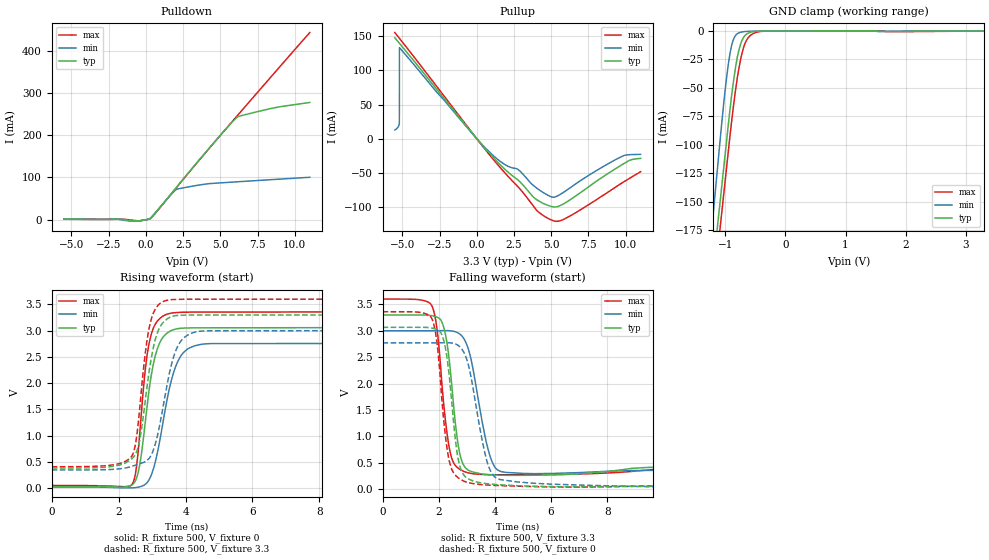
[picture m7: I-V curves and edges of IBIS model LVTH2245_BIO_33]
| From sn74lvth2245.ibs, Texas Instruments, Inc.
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[Model]   LVTH2245_BIO_33
Model_type  I/O
Vinl = 0.8
Vinh = 2.34
Enable   Active-Low
Vref =   0
Rref =   500
Cref =   50p
Vmeas =   1.5
| variable   typ   min   max
C_comp   6.47pF   5.20pF   8.54pF
| C_pullup   4.87pF   3.70pF   5.94pF
| C_pulldown   5.78pF   0.20pF   11.87pF
| C_tri-state   6.47pF   5.20pF   8.54pF
[Temperature Range]   40   -40   100
| Ambient temperature   25   -40   85
[Voltage range]   3.3   3   3.6
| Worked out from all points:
|   slope of the pulldown table from 0 to 0.495 V, typ, clamps not added: 47.8 ohm
|   slope of the pullup table from 0 to 0.495 V, typ, clamps not added: 38.7 ohm
|   GND clamp passes 1 mA (typ) near -0.58 V on its own axis
|   rising waveform, R_fixture 500, V_fixture 0: 20-80 % time 391ps typ, 525ps min, 307ps max; typ from 0.039 V to 3.06 V
|   falling waveform, R_fixture 500, V_fixture 3.3: 20-80 % time 348ps typ, 554ps min, 342ps max; typ from 3.3 V to 0.384 V
|   rising waveform, R_fixture 500, V_fixture 3.3: 20-80 % time 408ps typ, 518ps min, 335ps max; typ from 0.386 V to 3.3 V
|   falling waveform, R_fixture 500, V_fixture 0: 20-80 % time 365ps typ, 582ps min, 358ps max; typ from 3.07 V to 0.039 V
[GND Clamp]
| LVTH2245_BIO_33
|   Voltage   I(typ)   I(min)   I(max)
-5.5V     -2.567A    -2.796A    -2.574A
-1.235V   -223.4mA   -179.6mA   -246.1mA
-1.21V    -211mA     -165.3mA   -233.7mA
-1.155V   -183.6mA   -134mA     -206.5mA
-1.075V   -143.9mA   -88.81mA   -167mA
-975mV    -94.22mA   -38.79mA   -117.6mA
-900mV    -58.58mA   -13.51mA   -81.28mA
-825mV    -30mA      -3.451mA   -49.65mA
-775mV    -16.76mA   -1.557mA   -32.85mA
-650mV    -2.791mA   -308.1uA   -8.286mA
-375mV    -90.03uA   -77.36uA   -177.9uA
3.3V      36.14pA    29.2pA     -1.136uA
[Pulldown]
| LVTH2245_BIO_33
|   Voltage   I(typ)   I(min)   I(max)
-5.5V     1mA        970uA      796uA
-2V       861.7uA    1.289mA    689.4uA
-685mV    -3.317mA   -4.037mA   -2.363mA
-340mV    -2.425mA   -2.292mA   -2.574mA
315mV     3.262mA    4.023mA    3.242mA
1.715V    62.03mA    60.37mA    61.41mA
2.07V     77.36mA    72.02mA    76.76mA
4.09V     162.7mA    84.59mA    162.3mA
5.535V    221.5mA    88.27mA    221.9mA
6.12V     242.7mA    89.6mA     245.8mA
8.645V    265.1mA    95.2mA     348.5mA
11V       277.7mA    100.3mA    443.4mA
[Pullup]
| LVTH2245_BIO_33
|   Voltage   I(typ)   I(min)   I(max)
-5.5V     147.9mA    12.82mA    155.6mA
-5.195V   139.9mA    23.72mA    147.2mA
-5.19V    139.8mA    133.6mA    147.1mA
705mV     -18.04mA   -16.38mA   -19.55mA
1.825V    -43.56mA   -37.05mA   -48.54mA
2.81V     -61.39mA   -45.75mA   -71.52mA
3.835V    -86.3mA    -69.15mA   -99.73mA
4.695V    -97.03mA   -81.9mA    -115.7mA
5.185V    -100mA     -85.73mA   -120.5mA
5.865V    -95.04mA   -77.99mA   -117.9mA
9.65V     -39.48mA   -26.97mA   -66.25mA
11V       -28.86mA   -22.96mA   -48.42mA
[Ramp]
| LVTH2245_BIO_33
| variable   typ   min   max
dV/dt_r   1.82/4.00E-10   1.65/5.32E-10   2.00/3.13E-10
dV/dt_f   1.82/3.73E-10   1.63/5.73E-10   2.00/3.68E-10
R_load = 500
[Rising Waveform]
| LVTH2245_BIO_33
R_fixture =   500
C_fixture =   0
L_fixture =   0
V_fixture =   0
V_fixture_min = 0
V_fixture_max = 0
|   Time   V(typ)   V(min)   V(max)
0s        38.91mV    23.25mV    53.57mV
2.4ns     64.74mV    8.201mV    73.98mV
2.63ns    447mV      27.85mV    1.033V
2.795ns   1.25V      74.23mV    2.247V
2.94ns    2.006V     200.4mV    2.842V
3.215ns   2.749V     856.8mV    3.222V
3.655ns   3.021V     2.227V     3.34V
4.04ns    3.051V     2.641V     3.352V
4.76ns    3.054V     2.754V     3.354V
50ns      3.058V     2.757V     3.357V
[Falling Waveform]
| LVTH2245_BIO_33
R_fixture =   500
C_fixture =   0
L_fixture =   0
V_fixture =   3.3
V_fixture_min = 3
V_fixture_max = 3.6
|   Time   V(typ)   V(min)   V(max)
0s        3.3V       3V         3.6V
1.705ns   3.29V      3.001V     3.514V
1.91ns    3.264V     3.001V     3.148V
2.08ns    3.199V     3.002V     2.241V
2.465ns   1.972V     2.997V     584.8mV
2.77ns    629mV      2.931V     369.4mV
3.265ns   317.7mV    2.151V     288.3mV
3.835ns   271.1mV    616.1mV    272.3mV
4.39ns    261.1mV    316.1mV    270.1mV
50ns      384.5mV    346mV      408.8mV
[Rising Waveform]
| LVTH2245_BIO_33
R_fixture =   500
C_fixture =   0
L_fixture =   0
V_fixture =   3.3
V_fixture_min = 3
V_fixture_max = 3.6
|   Time   V(typ)   V(min)   V(max)
0s        385.7mV    348.6mV    409.6mV
2.39ns    560mV      416.5mV    605.7mV
2.625ns   907.4mV    467.2mV    1.487V
2.795ns   1.658V     506.8mV    2.566V
2.95ns    2.379V     605.1mV    3.155V
3.185ns   3.001V     1.075V     3.487V
3.545ns   3.257V     2.268V     3.588V
3.9ns     3.295V     2.832V     3.597V
4.61ns    3.297V     2.997V     3.599V
50ns      3.3V       3V         3.6V
[Falling Waveform]
| LVTH2245_BIO_33
R_fixture =   500
C_fixture =   0
L_fixture =   0
V_fixture =   0
V_fixture_min = 0
V_fixture_max = 0
|   Time   V(typ)   V(min)   V(max)
0s        3.066V     2.77V      3.361V
1.7ns     3.057V     2.771V     3.277V
1.905ns   3.03V      2.772V     2.906V
2.07ns    2.969V     2.772V     2.009V
2.45ns    1.736V     2.769V     396.5mV
2.75ns    442.4mV    2.698V     192.9mV
3.34ns    137.3mV    1.545V     95.62mV
3.945ns   90.95mV    262.6mV    70.87mV
5.38ns    53.91mV    110.5mV    46.39mV
50ns      38.81mV    23.19mV    53.65mV
